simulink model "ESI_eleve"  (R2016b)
settings: Solver=VariableStepAuto  StartTime=0.0  StopTime=inf  RelTol=1e-3
libraries: realtime_pacer_lib x1

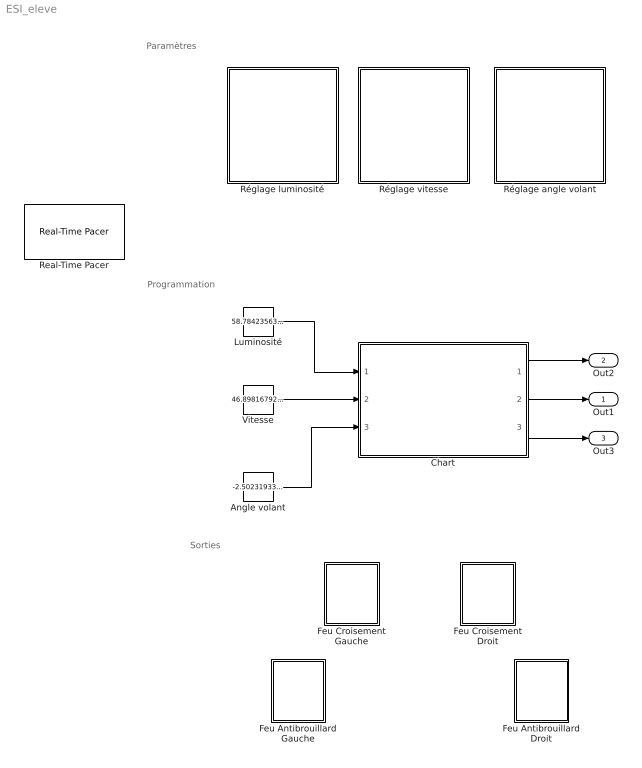
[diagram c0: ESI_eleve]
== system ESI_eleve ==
  note: Programmation
  note: Sorties
  note: Paramètres
  Angle volant : Constant  Value=-2.502319335938
  Chart : Stateflow chart  TreatAsAtomicUnit=on
  Feu Antibrouillard Droit : Subsystem  DialogController=hmiCreateDDGDialog  IsWebBlock=on
  Feu Antibrouillard Gauche : Subsystem  DialogController=hmiCreateDDGDialog  IsWebBlock=on
  Feu Croisement Droit : Subsystem  DialogController=hmiCreateDDGDialog  IsWebBlock=on
  Feu Croisement Gauche : Subsystem  DialogController=hmiCreateDDGDialog  IsWebBlock=on
  Luminosité : Constant  Value=58.784235636393
  Real-Time Pacer : realtime_pacer_lib/Real-Time Pacer  simTimePerRealTime=1
  Réglage angle volant : Subsystem  DialogController=hmiCreateDDGDialog  IsWebBlock=on
  Réglage luminosité : Subsystem  DialogController=hmiCreateDDGDialog  IsWebBlock=on
  Réglage vitesse : Subsystem  DialogController=hmiCreateDDGDialog  IsWebBlock=on
  Vitesse : Constant  Value=46.89816792806
  Out1 : Outport
  Out2 : Outport  Port=2
  Out3 : Outport  Port=3
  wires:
  Luminosité/1 -> Chart/1(luminosite)
  Vitesse/1 -> Chart/2(vitesse)
  Angle volant/1 -> Chart/3(angle)
  Chart/1(AB_G) -> Out2/1
  Chart/2(FC) -> Out1/1
  Chart/3(AB_D) -> Out3/1

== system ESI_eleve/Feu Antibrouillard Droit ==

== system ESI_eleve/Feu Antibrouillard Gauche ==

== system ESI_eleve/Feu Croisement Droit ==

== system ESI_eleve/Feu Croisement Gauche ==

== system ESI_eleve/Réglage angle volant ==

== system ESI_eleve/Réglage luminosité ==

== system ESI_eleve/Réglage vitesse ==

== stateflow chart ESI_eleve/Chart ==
  data: luminosite input; vitesse input; AB_G output; FC output; AB_D output; angle input
